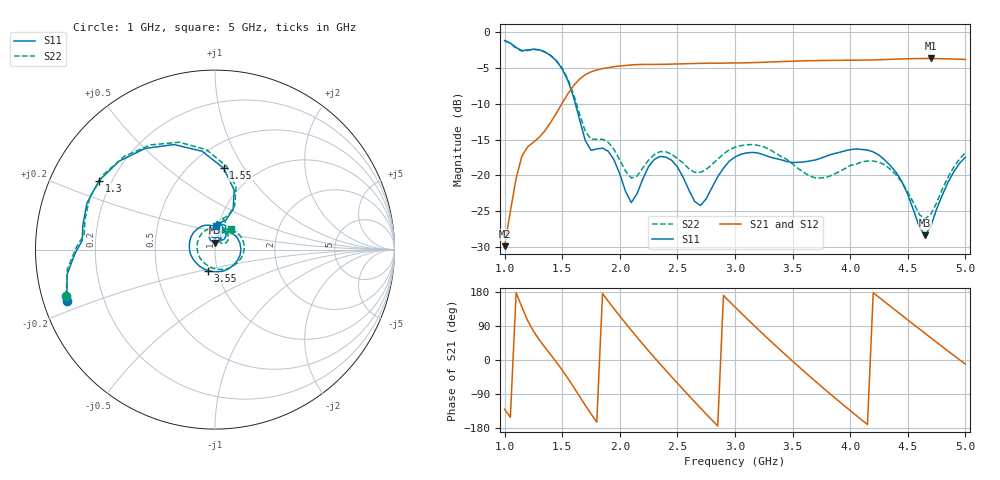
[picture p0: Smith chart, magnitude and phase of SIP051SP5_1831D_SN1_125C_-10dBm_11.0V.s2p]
# GHz  S  dB  R  50
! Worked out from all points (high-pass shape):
!   81 points, 1 GHz to 5 GHz, reference 50 ohm
!   highest |S21| = -3.69 dB at 4.7 GHz (marker M1); lowest = -29.9 dB at 1 GHz (marker M2)
!   |S21| within 3 dB of the highest: 1.643 GHz to end of sweep
!   lowest |S11| = -28.4 dB at 4.65 GHz (marker M3), VSWR 1.08, Z = 50 + j3.82 ohm
!   |S11| at or under -10 dB: 1.614 GHz to end of sweep
!   |S22| runs from -26.1 to -1.2 dB; largest |S21 - S12| = 0.0016
!   S11 on the Smith chart (normalised r, x): 1 GHz: 0.07, -0.17; 1.3 GHz: 0.15, +0.27; 1.55 GHz: 0.71, +0.82; 3.55 GHz: 0.90, -0.22; 5 GHz: 0.98, +0.27
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1  -1.18 -161.0  -29.86 -129.7  -29.93 -127.8  -1.22 -162.6
1.15  -2.60 176.1  -17.29 139.6  -17.30 139.8  -2.69 173.5
1.3  -2.48 149.2  -14.70 53.7  -14.69 53.7  -2.51 146.1
1.55  -6.81 84.0  -8.60 -48.6  -8.59 -48.6  -6.60 81.9
1.7  -15.13 69.6  -5.96 -119.3  -5.96 -119.2  -13.84 68.7
1.85  -16.20 84.3  -5.10 175.0  -5.11 175.2  -14.95 76.9
2.05  -22.24 73.0  -4.68 97.0  -4.66 97.0  -19.40 66.6
2.2  -20.48 109.5  -4.53 41.9  -4.53 41.9  -18.94 88.0
2.35  -17.35 87.5  -4.51 -10.6  -4.50 -10.6  -16.68 74.5
2.5  -18.81 57.8  -4.46 -61.2  -4.46 -61.2  -17.63 54.8
2.65  -23.62 52.9  -4.39 -110.4  -4.39 -110.5  -19.58 52.6
2.85  -20.18 70.4  -4.36 -174.2  -4.35 -174.2  -17.74 53.9
3  -17.43 40.3  -4.33 139.9  -4.32 139.8  -16.06 34.7
3.25  -17.14 -25.9  -4.22 66.6  -4.22 66.6  -16.01 -10.3
3.55  -18.18 -107.6  -4.05 -16.6  -4.05 -16.7  -19.05 -81.1
3.7  -17.83 -143.3  -4.00 -56.7  -3.99 -56.7  -20.35 -132.0
3.85  -16.99 -175.8  -3.96 -95.6  -3.95 -95.6  -19.91 174.4
4.05  -16.30 142.1  -3.94 -145.9  -3.92 -145.9  -18.43 114.4
4.35  -18.65 83.0  -3.81 141.5  -3.82 141.5  -19.16 50.1
4.65  -28.36 87.6  -3.70 70.2  -3.70 70.2  -26.07 51.8
4.7  -27.08 107.0  -3.69 58.4  -3.70 58.4  -25.39 65.1
5  -17.47 87.4  -3.82 -10.9  -3.82 -10.9  -16.83 52.9
